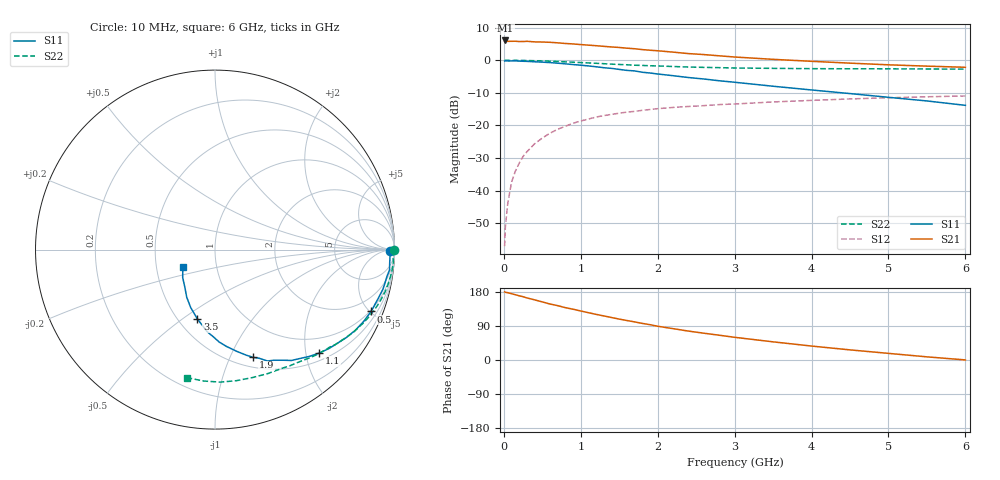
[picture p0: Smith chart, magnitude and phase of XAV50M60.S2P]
! SIEMENS Discrete & RF Semiconductors
! BFY180
! Si NPN RF Bipolar Junction Transistor in MICRO-X
! VCE = 0.5 V  IC = 0.6 mA
! Common Emitter S-Parameters:  May  1997
# GHz  S  MA  R  50
!  f  S11  S21  S12  S22
! GHz  MAG  ANG  MAG  ANG  MAG  ANG  MAG  ANG
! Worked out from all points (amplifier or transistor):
!   36 points, 10 MHz to 6 GHz, reference 50 ohm
!   highest |S21| = 6.1 dB at 20 MHz (marker M1)
!   |S21| within 3 dB of that: start of sweep to 1.9 GHz
!   unconditionally stable (mu >= 1): 3.066 GHz to end of sweep
!   at 250 MHz: K = 0.09, MSG = 17.6 dB, |S12| = -29.5 dB
!   at 1.4 GHz: K = 0.56, MSG = 10.4 dB, |S12| = -16.6 dB
!   at 6 GHz: K = 1.18, MAG = 1.9 dB, |S12| = -11.0 dB
!   S11 on the Smith chart (normalised r, x): 10 MHz: 74, -15; 500 MHz: 0.92, -5.08; 1.1 GHz: 0.65, -2.27; 1.9 GHz: 0.61, -1.23; 3.5 GHz: 0.62, -0.57; 6 GHz: 0.69, -0.14
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0.01  0.9745 -0.3  1.95 179.8  0.0014 81.8  0.9975 -0.2
0.02  0.9811 -0.9  2.013 178.8  0.0028 90.7  0.9999 -0.6
0.05  0.9759 -2.0  1.95 177.7  0.0062 89.7  0.9968 -1.4
0.1  0.9761 -4.3  1.955 175.0  0.0134 88.8  0.9935 -2.8
0.15  0.9791 -6.7  1.958 172.2  0.0199 84.7  0.9967 -4.3
0.25  0.9652 -11.1  1.938 167.0  0.0334 82.0  0.9929 -7.1
0.3  0.9613 -13.3  1.953 163.8  0.0394 80.4  0.9896 -8.5
0.5  0.9354 -21.6  1.904 153.3  0.064 73.4  0.9764 -13.9
0.6  0.9203 -25.7  1.885 147.7  0.0759 70.4  0.9666 -16.5
0.8  0.8802 -33.9  1.808 138.1  0.0972 64.0  0.9444 -21.6
1.1  0.8179 -44.8  1.706 124.8  0.1252 55.7  0.9096 -28.5
1.5  0.7236 -58.4  1.571 107.9  0.154 46.2  0.8615 -36.9
1.9  0.6374 -70.4  1.425 93.2  0.1754 38.7  0.8235 -43.8
2  0.6151 -73.3  1.398 89.1  0.1805 37.5  0.8172 -45.5
2.2  0.5793 -78.0  1.333 82.7  0.1888 33.9  0.8014 -48.8
2.4  0.5429 -83.3  1.265 76.3  0.1953 31.2  0.7875 -51.7
2.8  0.4844 -91.3  1.17 65.4  0.2087 26.6  0.77 -57.3
3.5  0.3991 -104.2  1.033 47.9  0.2291 19.5  0.7508 -66.9
4  0.3498 -112.8  0.963 36.8  0.2422 14.4  0.7428 -73.8
4.5  0.308 -120.8  0.903 26.7  0.2548 9.5  0.74 -80.8
5.5  0.2373 -139.4  0.812 8.3  0.2749 0.0  0.7349 -95.0
6  0.2032 -151.7  0.78 0.2  0.2829 -4.9  0.7301 -102.2
